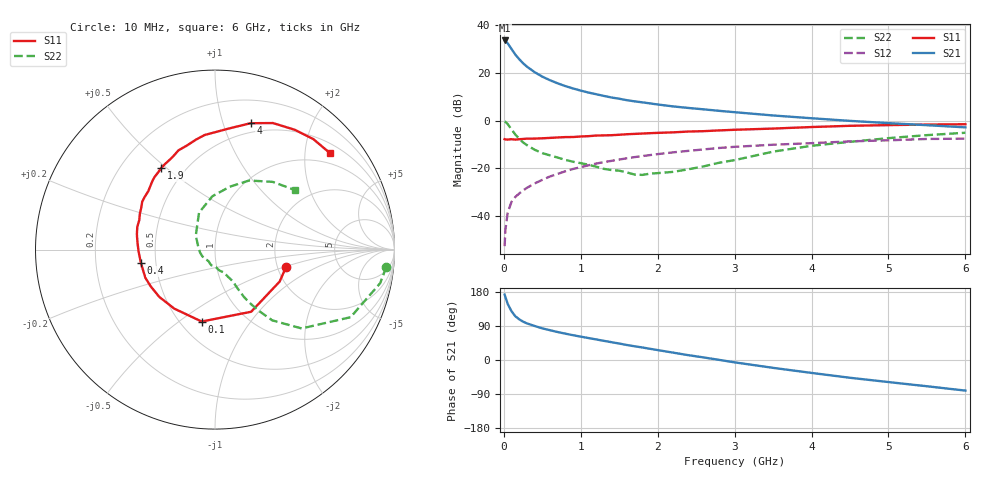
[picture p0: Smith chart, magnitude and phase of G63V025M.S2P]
! SIEMENS Small Signal Semiconductors
! BFG193
! Si NPN RF Bipolar Junction Transistor in SOT223
! VCE = 3 V  IC = 25 mA
! Common Emitter S-Parameters:  August  1996
# GHz  S  MA  R  50
!  f  S11  S21  S12  S22
! GHz  MAG  ANG  MAG  ANG  MAG  ANG  MAG  ANG
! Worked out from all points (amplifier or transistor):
!   36 points, 10 MHz to 6 GHz, reference 50 ohm
!   highest |S21| = 33.4 dB at 10 MHz (marker M1)
!   |S21| within 3 dB of that: start of sweep to 88.12 MHz
!   unconditionally stable (mu >= 1): 625.4 MHz to 2.523 GHz
!   at 250 MHz: K = 0.80, MSG = 26.5 dB, |S12| = -29.2 dB
!   at 1.4 GHz: K = 1.05, MAG = 11.8 dB, |S12| = -16.8 dB
!   at 6 GHz: K = 0.89, MSG = 2.4 dB, |S12| = -7.6 dB
!   S11 on the Smith chart (normalised r, x): 10 MHz: 2.24, -0.51; 100 MHz: 0.63, -0.61; 400 MHz: 0.41, -0.08; 1.9 GHz: 0.37, +0.48; 4 GHz: 0.41, +1.24; 6 GHz: 0.72, +2.57
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0.01  0.4078 -13.4  46.67 172.6  0.0024 86.9  0.9593 -5.8
0.02  0.4018 -26.3  45.79 166.5  0.0052 83.6  0.939 -11.5
0.05  0.4007 -59.8  40.62 148.1  0.012 71.4  0.8441 -26.5
0.1  0.4076 -100.5  30.98 128.6  0.0202 63.5  0.6527 -42.3
0.15  0.3996 -124.6  23.62 115.2  0.0256 59.6  0.5076 -51.0
0.2  0.4072 -139.6  19 107.4  0.0301 60.9  0.4173 -54.5
0.25  0.4126 -150.2  15.64 101.2  0.0348 61.1  0.3493 -57.2
0.3  0.4185 -157.9  13.29 96.6  0.0395 62.2  0.3073 -58.6
0.4  0.4195 -169.5  10.19 89.8  0.0487 62.6  0.2457 -59.9
0.5  0.426 -178.7  8.214 83.5  0.0579 62.7  0.2092 -60.6
0.6  0.4338 174.8  6.918 78.6  0.0681 62.4  0.1875 -62.0
0.7  0.4435 168.9  5.962 73.8  0.0772 61.8  0.1688 -64.4
0.9  0.4528 158.7  4.657 65.4  0.0977 59.1  0.1382 -68.3
1.1  0.4717 150.7  3.83 58.0  0.1164 56.3  0.1198 -77.8
1.4  0.494 138.8  3.016 47.0  0.1442 50.3  0.0927 -94.6
1.9  0.5445 123.4  2.275 29.6  0.1903 40.2  0.078 -140.1
2.2  0.5664 114.9  1.968 19.5  0.2169 33.3  0.085 -169.3
3.5  0.6793 83.4  1.274 -20.7  0.3127 2.6  0.2244 113.3
4  0.7314 74.3  1.115 -34.1  0.3373 -7.1  0.2972 92.9
4.5  0.7755 65.4  0.983 -46.9  0.3673 -17.2  0.3598 76.8
5.5  0.8242 48.3  0.799 -69.3  0.4125 -40.5  0.4956 49.6
6  0.8362 40.0  0.72 -80.7  0.4181 -53.8  0.5554 36.7
